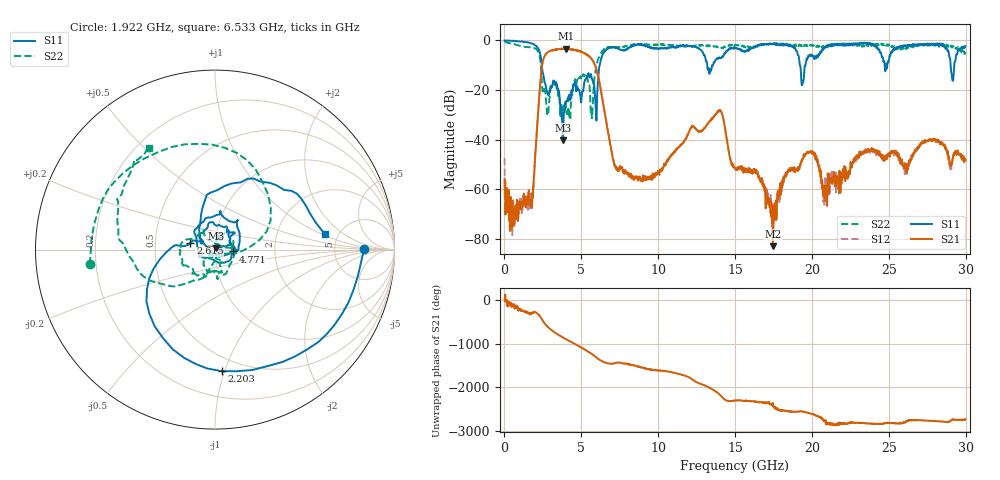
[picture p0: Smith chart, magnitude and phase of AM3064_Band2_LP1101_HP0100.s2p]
# Hz S DB R 50.0
!freq dBS11 angS11 dBS21 angS21 dBS12 angS12 dBS22 angS22
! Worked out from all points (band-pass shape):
!   1600 points, 10 MHz to 29.98 GHz, reference 50 ohm
!   highest |S21| = -3.35 dB at 4.002 GHz (marker M1); lowest = -83.0 dB at 17.46 GHz (marker M2)
!   |S21| within 3 dB of the highest: 2.613 GHz to 5.478 GHz (2.864 GHz wide, 70.8 % of centre)
!   lowest |S11| = -40.3 dB at 3.796 GHz (marker M3), VSWR 1.02, Z = 50.7 + j0.637 ohm
!   |S11| at or under -10 dB: 2.427 GHz to 6.193 GHz (3.767 GHz wide, 87.4 % of centre); 13.19 GHz to 13.56 GHz (374.4 MHz wide, 2.8 % of centre); 19.22 GHz to 19.58 GHz (357.5 MHz wide, 1.84 % of centre)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
!   |S22| runs from -32.1 to -0.2 dB; largest |S21 - S12| = 0.02
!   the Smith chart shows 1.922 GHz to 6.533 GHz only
!   S11 on the Smith chart (normalised r, x): 1.922 GHz: 11, +0; 2.203 GHz: 0.39, -0.98; 2.615 GHz: 0.76, +0.06; 4.771 GHz: 1.22, -0.03; 6.533 GHz: 3.90, +1.12
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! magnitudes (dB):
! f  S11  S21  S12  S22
! 10 MHz  -0.1  -56.0  -47.6  -0.2
! 609.8 MHz  -0.2  -70.0  -74.4  -1.5
! 1.922 GHz  -1.6  -55.1  -55.1  -3.1
! 2.203 GHz  -3.4  -27.9  -27.9  -4.7
! 2.615 GHz  -17.0  -6.3  -6.3  -20.5
! 3.796 GHz  -40.3  -3.4  -3.4  -29.1
! 4.002 GHz  -24.6  -3.4  -3.4  -27.5
! 4.771 GHz  -19.9  -4.2  -4.1  -16.5
! 5.015 GHz  -23.0  -4.6  -4.6  -15.7
! 5.689 GHz  -15.4  -7.6  -7.7  -31.4
! 5.952 GHz  -28.4  -11.0  -11.0  -11.0
! 6.533 GHz  -4.2  -29.5  -29.4  -3.4
! 7.301 GHz  -3.1  -51.8  -51.8  -2.7
! 10 GHz  -3.4  -53.6  -53.5  -1.8
! 13.97 GHz  -6.9  -28.6  -28.3  -2.9
! 15 GHz  -2.9  -51.7  -51.6  -1.9
! 17.46 GHz  -1.3  -83.0  -74.8  -1.3
! 19.37 GHz  -17.8  -47.9  -48.2  -2.0
! 19.99 GHz  -5.8  -45.0  -45.5  -1.9
! 20.83 GHz  -3.2  -58.8  -62.7  -2.3
! 25 GHz  -8.1  -45.8  -45.8  -1.7
! 29.98 GHz  -2.3  -48.3  -48.5  -4.7
